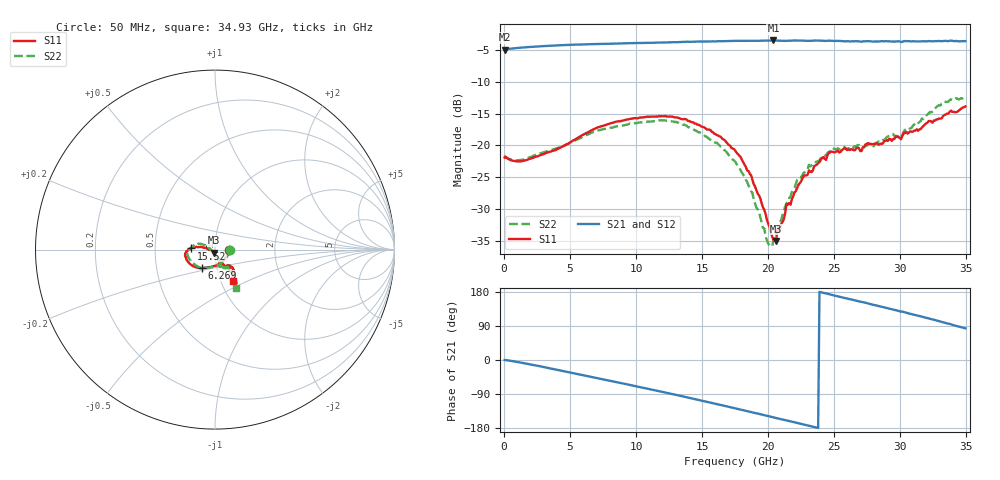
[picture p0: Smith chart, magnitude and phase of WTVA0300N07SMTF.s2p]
! 50 ohm 2-Port S-parameters measured by Modelithics Inc support@modelithics.com  Tampa, FL USA 813-866-6335 (February 2024)
! Smiths Interconnect,  3dB P/N: WTVA0300N07SMTF, Temperature: -25 C
! Board: 10 mil Rogers 4350B, Mounting Pad Dimensions: Length: 15 mils, Width: 25 mils, Gap: 40 mils.
# Hz S RI R 50
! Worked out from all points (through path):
!   352 points, 50 MHz to 34.93 GHz, reference 50 ohm
!   highest |S21| = -3.57 dB at 20.4 GHz (marker M1); lowest = -5.0 dB at 50 MHz (marker M2)
!   group delay of S21, straight-line fit = 22.1 ps
!   lowest |S11| = -34.9 dB at 20.6 GHz (marker M3), VSWR 1.04, Z = 49.2 - j1.6 ohm
!   |S11| at or under -10 dB: start of sweep to end of sweep
!   |S22| runs from -35.8 to -12.4 dB; largest |S21 - S12| = 0.0064
!   S11 on the Smith chart (normalised r, x): 50 MHz: 1.17, -0.01; 6.269 GHz: 0.85, -0.18; 15.52 GHz: 0.77, +0.01; 34.93 GHz: 1.14, -0.42
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5e7  0.0804 -0.00344  0.5626 -0.000425  0.562 -0.000532  0.0835 -0.00331
1.593e9  0.0474 -0.0599  0.5787 -0.0911  0.5781 -0.0911  0.0487 -0.0614
5.8715e9  -0.0617 -0.1025  0.4791 -0.3882  0.4784 -0.3883  -0.0553 -0.1014
6.2695e9  -0.0727 -0.1026  0.4604 -0.4132  0.4595 -0.4134  -0.0661 -0.1014
1.1742e10  -0.165 -0.0411  0.0845 -0.6315  0.0829 -0.6312  -0.1535 -0.0334
1.5523e10  -0.1329 0.0062  -0.2406 -0.6047  -0.2418 -0.6036  -0.1098 0.0264
1.7513e10  -0.0897 0.015  -0.4021 -0.5209  -0.4032 -0.5194  -0.0683 0.0294
1.88065e10  -0.0529 0.00994  -0.4919 -0.4392  -0.4925 -0.4378  -0.0396 0.0155
2.00005e10  -0.0237 -0.00624  -0.5614 -0.3507  -0.5615 -0.3499  -0.0158 -0.00661
2.03985e10  -0.0137 -0.0119  -0.582 -0.3173  -0.5825 -0.3155  -0.00835 -0.0158
2.05975e10  -0.00753 -0.0163  -0.5896 -0.2994  -0.5902 -0.297  -0.00568 -0.0203
2.0697e10  -0.00746 -0.0207  -0.5935 -0.2908  -0.5941 -0.2885  -0.00441 -0.021
2.11945e10  0.0012 -0.0267  -0.6098 -0.248  -0.61 -0.2462  0.00472 -0.0306
2.13935e10  0.0037 -0.0346  -0.6154 -0.2323  -0.6157 -0.2303  0.0056 -0.0349
2.1692e10  0.00618 -0.0339  -0.6282 -0.2068  -0.6282 -0.205  0.0115 -0.0382
2.21895e10  0.0157 -0.0439  -0.6416 -0.1578  -0.6415 -0.1556  0.018 -0.0504
2.33835e10  0.0241 -0.0593  -0.6585 -0.0492  -0.6582 -0.0478  0.0243 -0.0668
2.45775e10  0.0338 -0.0811  -0.6571 0.0697  -0.6565 0.0716  0.0287 -0.0841
2.91545e10  0.0592 -0.096  -0.4652 0.4576  -0.4629 0.4592  0.0568 -0.1044
3.01495e10  0.0806 -0.087  -0.397 0.5095  -0.3949 0.5107  0.0704 -0.0964
3.2239e10  0.0993 -0.1199  -0.211 0.6212  -0.2103 0.6209  0.1057 -0.1491
3.49255e10  0.1014 -0.1745  0.0733 0.6509  0.0783 0.6498  0.115 -0.2112
